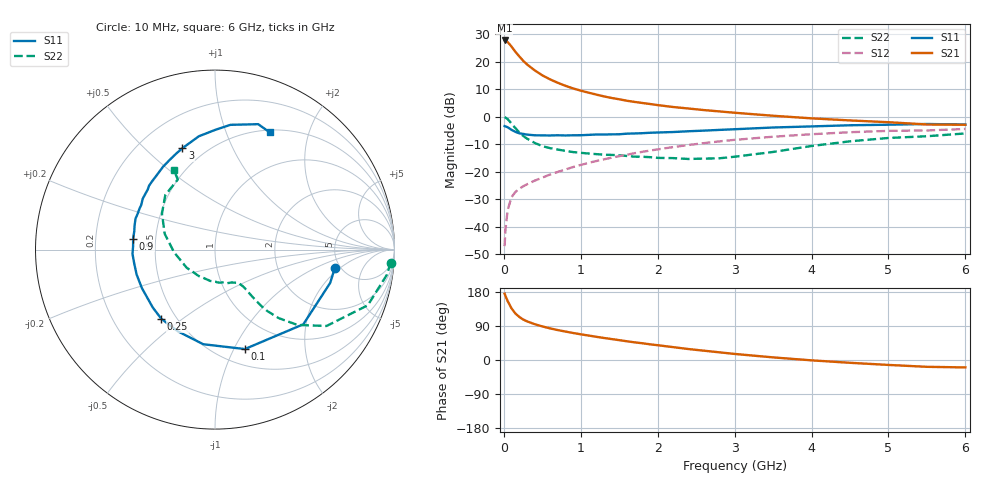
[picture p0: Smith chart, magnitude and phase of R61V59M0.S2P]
! SIEMENS Small Signal Semiconductors
! BFR193
! Si NPN RF Bipolar Junction Transistor in SOT23
! VCE = 1.5 V  IC = 9 mA
! Common Emitter S-Parameters:  May  1996
# GHz  S  MA  R  50
!  f  S11  S21  S12  S22
! GHz  MAG  ANG  MAG  ANG  MAG  ANG  MAG  ANG
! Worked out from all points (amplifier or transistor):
!   36 points, 10 MHz to 6 GHz, reference 50 ohm
!   highest |S21| = 27.8 dB at 10 MHz (marker M1)
!   |S21| within 3 dB of that: start of sweep to 120.4 MHz
!   unconditionally stable (mu >= 1): 737.9 MHz to 2.033 GHz
!   at 250 MHz: K = 0.62, MSG = 22.9 dB, |S12| = -25.4 dB
!   at 1.4 GHz: K = 1.05, MAG = 9.5 dB, |S12| = -14.9 dB
!   at 6 GHz: K = 0.96, MSG = 0.8 dB, |S12| = -4.4 dB
!   S11 on the Smith chart (normalised r, x): 10 MHz: 4.53, -1.66; 100 MHz: 0.66, -1.11; 250 MHz: 0.41, -0.42; 900 MHz: 0.37, +0.06; 3 GHz: 0.38, +0.66; 6 GHz: 0.53, +1.43
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0.01  0.6756 -8.5  24.54 174.9  0.0044 86.8  0.9826 -4.2
0.02  0.6682 -16.1  24.11 169.6  0.0085 80.6  0.9673 -8.4
0.05  0.6445 -40.2  22.93 155.2  0.0201 72.9  0.9062 -20.0
0.1  0.5785 -73.3  18.99 136.2  0.0344 60.9  0.7532 -34.4
0.15  0.5312 -97.1  15.28 122.7  0.0426 55.5  0.6226 -42.4
0.2  0.5002 -114.4  12.62 113.8  0.0488 53.8  0.5209 -47.1
0.25  0.488 -127.8  10.53 107.0  0.054 52.9  0.4492 -49.6
0.3  0.4735 -137.1  9.011 102.1  0.0588 53.3  0.4016 -50.7
0.4  0.4603 -152.3  7.025 94.6  0.0686 55.0  0.3349 -51.6
0.5  0.4582 -162.3  5.694 88.6  0.0779 56.9  0.2919 -52.0
0.6  0.4566 -170.3  4.803 83.5  0.0886 58.2  0.2684 -52.4
0.7  0.4604 -177.0  4.168 79.0  0.0989 59.5  0.2527 -53.0
0.9  0.4601 172.3  3.286 71.3  0.1214 60.7  0.2276 -55.0
1.1  0.4682 163.1  2.751 64.6  0.1445 61.0  0.2143 -59.3
1.3  0.4748 155.4  2.353 58.2  0.1678 60.2  0.2039 -63.8
1.6  0.4925 144.8  1.958 49.4  0.2041 58.3  0.1932 -73.3
2.2  0.5274 127.7  1.507 34.0  0.2802 52.4  0.1767 -98.6
3  0.5931 107.9  1.184 16.0  0.3802 41.5  0.1873 -147.2
3.5  0.6378 98.1  1.044 6.9  0.4333 33.7  0.2286 -176.3
4.5  0.7006 82.9  0.858 -7.4  0.5233 18.5  0.3572 145.8
5.5  0.7391 71.0  0.724 -18.0  0.5637 3.2  0.4423 118.0
6  0.7212 65.1  0.715 -19.6  0.5999 -1.3  0.4973 117.3
